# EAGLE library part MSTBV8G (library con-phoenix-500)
PHOENIX
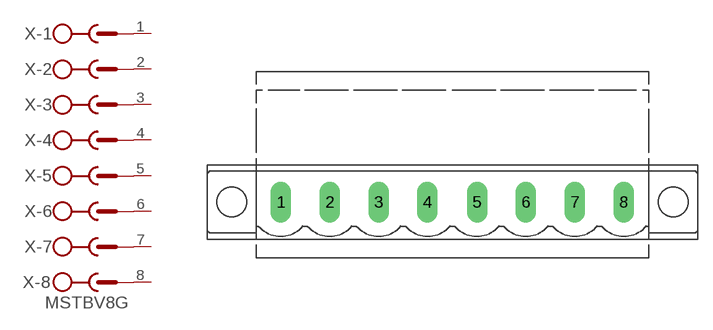
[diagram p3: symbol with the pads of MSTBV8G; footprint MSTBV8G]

Designator prefix X; gates -1=SK -2=SK -3=SK -4=SK -5=SK -6=SK -7=SK -8=SK+V

## MSTBV8G (OC_FARNELL: unknown; OC_NEWARK: unknown)  [MSTBV8G]
1  -1:SK  pas
2  -2:SK  pas
3  -3:SK  pas
4  -4:SK  pas
5  -5:SK  pas
6  -6:SK  pas
7  -7:SK  pas
8  -8:SK  pas

## Footprint MSTBV8G (pad centres in mm)
PHOENIX
drill 1.397 long: 1 -17.5,0; 2 -12.522,0; 3 -7.518,0; 4 -2.565,0; 5 2.515,0; 6 7.494,0; 7 12.497,0; 8 17.501,0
